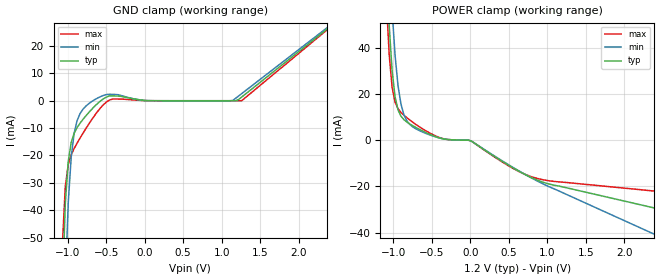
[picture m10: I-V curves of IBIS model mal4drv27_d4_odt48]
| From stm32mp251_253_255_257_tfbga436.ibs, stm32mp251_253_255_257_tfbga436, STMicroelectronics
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[Model] mal4drv27_d4_odt48
Model_type   Input
Polarity   Non-Inverting
Enable   Active-High
C_comp   2.040pF   1.736pF   2.110pF
C_comp_power_clamp   988.438fF   798.145fF   1.019pF
C_comp_gnd_clamp 896.306fF   838.028fF   922.296fF
Vinh = 879.000mV
Vinl = 764.000mV
[Model Spec]
D_overshoot_ampl_h 0.24 NA   NA
D_overshoot_ampl_l 0.24 NA   NA
D_overshoot_area_l 300.000m NA   NA
D_overshoot_area_h 300.000m NA   NA
[Receiver Thresholds]
Vth = 821.000mV
Vth_min = 780.000mV
Vth_max = 862.000mV
Vinh_ac = 68.000mV
Vinh_dc = 68.000mV
Vinl_ac = -68.000mV
Vinl_dc = -68.000mV
Tslew_ac = 5.000ns
Threshold_sensitivity = 0.5
Reference_supply Power_clamp_ref
[Temperature Range]   25.000   125.000   -40.000
[Voltage Range]   1.200V   1.140V   1.260V
[GND Clamp Reference]   0.00V   0.00V   0.00V
[C Comp Corner]
| variable   typ   min   max
C_comp 2.040pF   1.736pF   2.110pF
C_comp_pullup 988.438fF   798.145fF   1.019pF
C_comp_pulldown 896.306fF   838.028fF   922.296fF
[POWER Clamp Reference]   1.200V   1.140V   1.260V
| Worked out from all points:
|   GND clamp passes 1 mA (typ) near -0.20 V on its own axis
|   POWER clamp passes 1 mA (typ) near -0.40 V on its own axis
[GND Clamp]
-1.184V   -305.9mA   -358.6mA   -282.9mA
-1.069V   -69.76mA   -112.9mA   -52.66mA
-1.031V   -37.56mA   -66.48mA   -31.37mA
-992.7mV  -22.16mA   -37.24mA   -23.33mA
-954.6mV  -15.27mA   -20.7mA    -19.77mA
-916.4mV  -11.89mA   -11.93mA   -17.47mA
-840mV    -8.234mA   -4.712mA   -13.68mA
-725.5mV  -4.29mA    -1.06mA    -8.5mA
-420mV    1.759mA    2.326mA    628uA
1.145V    448nA      108.1uA    23.65nA
1.26V     1.339mA    2.595mA    27.75nA
2.367V    26.17mA    26.63mA    25.85mA
[Power Clamp]
-1.167V   155.7mA    192.5mA    138.3mA
-1.091V   78.34mA    114.4mA    61.8mA
-1.053V   49.77mA    82.25mA    37.1mA
-1.015V   30.07mA    56.14mA    22.95mA
-976.4mV  18.76mA    36.72mA    16.46mA
-938.2mV  13.15mA    23.64mA    13.62mA
-900mV    10.42mA    15.64mA    12.03mA
-785.5mV  7.05mA     6.845mA    8.761mA
-403.6mV  1.024mA    1.026mA    1.233mA
16.36mV   -373.8uA   -406.6uA   -387.7uA
856.4mV   -17.05mA   -17.38mA   -16.4mA
2.384V    -29.22mA   -40.53mA   -21.95mA
